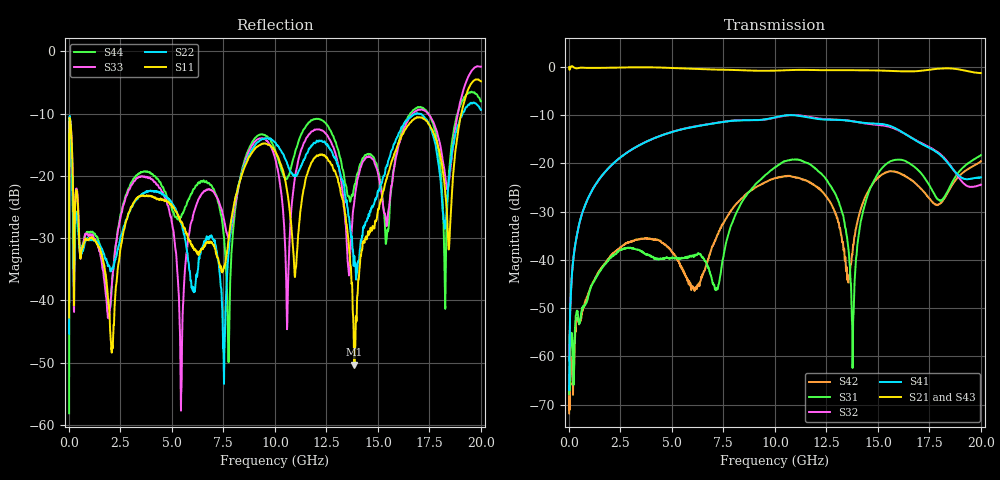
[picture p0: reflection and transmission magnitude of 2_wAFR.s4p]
!Keysight Technologies,N5225A,MY51451420,A.10.40.12
!Date: Tuesday, October 13, 2015 10:20:41
!Correction: S11(Full 4 Port(1,2,3,4))
!S12(Full 4 Port(1,2,3,4))
!S13(Full 4 Port(1,2,3,4))
!S14(Full 4 Port(1,2,3,4))
!S21(Full 4 Port(1,2,3,4))
!S22(Full 4 Port(1,2,3,4))
!S23(Full 4 Port(1,2,3,4))
!S24(Full 4 Port(1,2,3,4))
!S31(Full 4 Port(1,2,3,4))
!S32(Full 4 Port(1,2,3,4))
!S33(Full 4 Port(1,2,3,4))
!S34(Full 4 Port(1,2,3,4))
!S41(Full 4 Port(1,2,3,4))
!S42(Full 4 Port(1,2,3,4))
!S43(Full 4 Port(1,2,3,4))
!S44(Full 4 Port(1,2,3,4))
!S4P File: Measurements: <S11,S12,S13,S14>,
!<S21,S22,S23,S24>,
!<S31,S32,S33,S34>,
!<S41,S42,S43,S44>:
# Hz S  dB  R 50
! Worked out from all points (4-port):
!   2000 points, 10 MHz to 20 GHz, reference 50 ohm
!   strongest paths, dB at 10 MHz, 5.01 GHz, 10.01 GHz, 15.01 GHz, 20 GHz:
!     S21: 0.0, -0.2, -0.7, -0.7, -1.2
!     S43: -0.1, -0.2, -0.7, -0.7, -1.8
!     S41: -67.0, -13.5, -10.4, -11.7, -22.9
!     S32: -60.8, -13.4, -10.5, -12.0, -24.4
!     S31: -67.9, -39.5, -20.8, -22.1, -18.3
!     S42: -71.8, -38.4, -23.0, -22.9, -19.5
!   lowest |S11| = -50.3 dB at 13.86 GHz (marker M1), VSWR 1.01, Z = 49.8 - j0.256 ohm
!   |S11| at or under -10 dB: start of sweep to 19.05 GHz
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1e7  -42.76 -27.5  -0.01 0.3  -81.71 -128.5  -74.16 128.0
     -0.02 0.4  -45.35 162.0  -61.22 81.4  -74.45 39.5
     -67.87 153.5  -60.78 102.6  -40.21 -15.8  -0.07 0.6
     -66.96 67.7  -71.82 170.9  -0.07 0.1  -58.14 176.1
4.7e8  -27.52 63.5  -0.18 0.4  -52.65 117.0  -33.14 90.7
       -0.18 0.4  -29.54 79.4  -33.15 90.6  -52.73 122.0
       -52.64 115.9  -33.14 90.3  -26.91 67.2  -0.19 0.4
       -33.12 90.3  -52.70 119.1  -0.17 0.4  -28.85 80.1
2.26e9  -38.72 -170.9  -0.11 8.4  -38.75 35.6  -19.58 98.5
        -0.12 8.5  -33.46 -98.8  -19.58 98.0  -38.21 131.0
        -38.76 35.8  -19.59 98.0  -31.35 -159.0  -0.14 8.5
        -19.59 98.6  -38.18 130.8  -0.12 8.5  -31.32 -67.2
7.52e9  -34.82 45.6  -0.55 33.5  -38.84 -55.4  -11.35 125.1
        -0.55 33.8  -51.23 -7.8  -11.32 122.9  -32.24 -74.4
        -38.77 -55.4  -11.33 122.8  -26.84 14.1  -0.58 34.3
        -11.35 125.3  -32.26 -74.6  -0.56 34.4  -29.52 -89.1
9.53e9  -14.78 82.8  -0.76 35.3  -22.39 155.3  -10.83 129.3
        -0.77 35.7  -13.94 171.7  -10.86 126.0  -23.90 -136.7
        -22.40 155.4  -10.87 125.8  -14.09 100.9  -0.81 36.5
        -10.84 129.5  -23.89 -136.8  -0.80 36.6  -13.47 160.4
1.386e10  -50.34 -122.4  -0.65 64.5  -45.60 40.3  -11.30 158.5
          -0.65 65.0  -32.87 -150.2  -11.29 153.0  -35.09 -27.5
          -45.67 40.6  -11.29 152.8  -23.99 35.6  -0.70 66.0
          -11.30 159.0  -35.03 -27.9  -0.68 66.3  -21.46 -112.5
2e10  -4.79 -123.0  -1.22 89.1  -18.26 -113.7  -22.87 -133.9
      -1.23 89.7  -9.40 177.8  -24.38 -130.9  -19.57 128.6
      -18.27 -113.6  -24.40 -131.5  -2.45 -113.6  -1.81 92.7
      -22.88 -133.2  -19.54 128.4  -1.80 93.0  -8.03 156.9
